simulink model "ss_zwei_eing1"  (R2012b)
settings: Solver=ode45  StartTime=0.0  StopTime=100  RelTol=1e-3
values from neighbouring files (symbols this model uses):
  dt = 0.01    [aktiv_tilger_1.m]    (also in aktiv_tilger_12.m; aktiv_tilger_2.m; beobachter_1.m; beobachter_2.m)
  Kest = kalman(P,1,0.01),    [LQG_1.m]    (also in ss_zwei_eing_1.m = kalman(sys2, Q, R))
  sys2 = sys1(:,[1,1,1])    [kalman_11.m]    (also in kalman_12.m; kalman_13.m = sys1(:,[1,1,1,1]); kalman_2.m = ss(H2); kalman_3.m = ss(H2))
  vnd = 1e-4    (= 0.0001)    [kalman_1.m]    (also in kalman_10.m; kalman_11.m; kalman_12.m; kalman_13.m = 0.01)
  vny = 1e-6    (= 1e-06)    [kalman_1.m]    (also in kalman_10.m; kalman_11.m = ', num2str(vny),' )']); kalman_12.m = ', num2str(vny),' )']); kalman_13.m = ', num2str(vny),' )']))
libraries: simulink x2

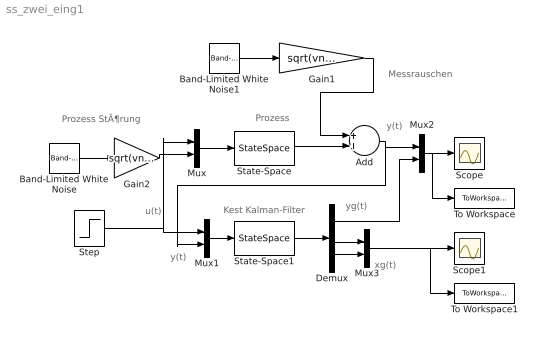
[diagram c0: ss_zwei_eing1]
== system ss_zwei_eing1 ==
  note: y(t)
  note: xg(t)
  note: u(t)
  note: y(t)
  note: yg(t)
  note: Messrauschen
  note: Prozess StÃ¶rung
  note: Kest Kalman-Filter
  note: Prozess
  Add : Sum
  Band-Limited White Noise : simulink/Sources/Band-Limited White Noise  Cov=[dt, dt]  Ts=dt  seed=[23341, 2785]
  Band-Limited White Noise1 : simulink/Sources/Band-Limited White Noise  Cov=dt  Ts=dt  seed=[23341]
  Demux : Demux  Outputs=3
  Gain1 : Gain  Gain=sqrt(vny)
  Gain2 : Gain  Gain=sqrt(vnd)*eye(2,2)  Multiplication=Matrix(K*u)
  Mux{,1..3} (4 alike) : Mux  Inputs=2
  Scope : Scope
  Scope1 : Scope
  State-Space : StateSpace  A=sys2.a  B=sys2.b  C=sys2.c  D=sys2.d
  State-Space1 : StateSpace  A=Kest.a  B=Kest.b  C=Kest.c  D=Kest.d
  Step : Step  SampleTime=0
  To Workspace : ToWorkspace  VariableName=y  SampleTime=-1  SaveFormat=Structure With Time
  To Workspace1 : ToWorkspace  VariableName=y1  SampleTime=-1  SaveFormat=Structure With Time
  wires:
  Mux/1 -> State-Space/1
  Band-Limited White Noise/1 -> Gain2/1
  Step/1 -> Mux/1, Mux1/1
  Gain2/1 -> Mux/2
  Band-Limited White Noise1/1 -> Gain1/1
  State-Space/1 -> Add/2
  Gain1/1 -> Add/1
  Add/1 -> Mux1/2, Mux2/1
  Mux1/1 -> State-Space1/1
  State-Space1/1 -> Demux/1
  Mux2/1 -> To Workspace/1, Scope/1
  Demux/1 -> Mux2/2
  Demux/2 -> Mux3/1
  Demux/3 -> Mux3/2
  Mux3/1 -> To Workspace1/1, Scope1/1
